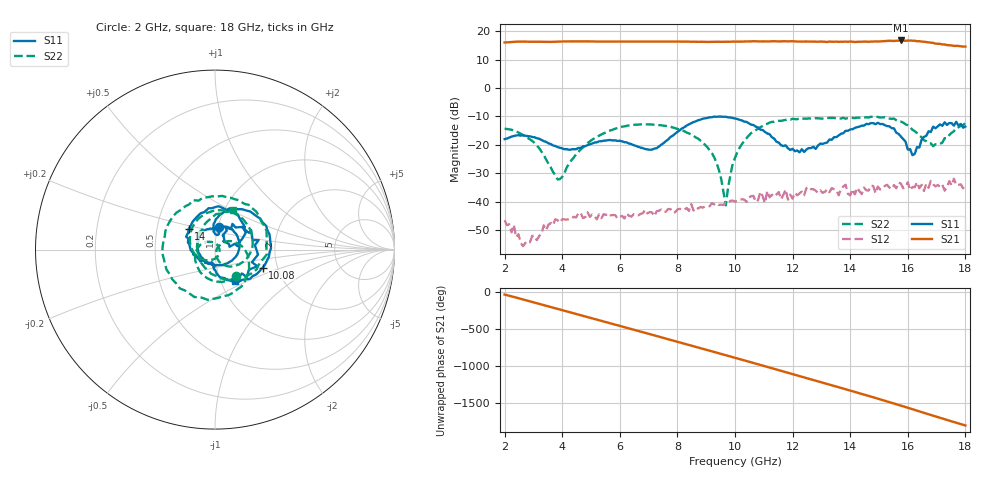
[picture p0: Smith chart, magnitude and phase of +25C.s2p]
!Agilent Technologies,N5230A,MY45001466,A.07.50.67
!Agilent N5230A: A.07.50.67
!Date: Monday, February 09, 2026 16:21:58
!Correction: S11(Full 2 Port(1,2))
!S21(Full 2 Port(1,2))
!S12(Full 2 Port(1,2))
!S22(Full 2 Port(1,2))
!S2P File: Measurements: S11, S21, S12, S22:
# Hz S  dB  R 50
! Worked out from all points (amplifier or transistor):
!   201 points, 2 GHz to 18 GHz, reference 50 ohm
!   highest |S21| = 16.7 dB at 15.76 GHz (marker M1)
!   |S21| within 3 dB of that: start of sweep to end of sweep
!   unconditionally stable (mu >= 1): start of sweep to end of sweep
!   at 4.64 GHz: K = 11.69, MAG = 16.5 dB, |S12| = -43.9 dB
!   at 10 GHz: K = 6.99, MAG = 16.7 dB, |S12| = -40.0 dB
!   at 18 GHz: K = 4.16, MAG = 15.1 dB, |S12| = -33.9 dB
!   S11 on the Smith chart (normalised r, x): 2 GHz: 1.01, +0.26; 10.08 GHz: 1.67, -0.37; 14 GHz: 0.73, +0.17; 18 GHz: 1.17, -0.43
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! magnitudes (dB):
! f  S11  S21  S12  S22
! 2 GHz  -18.0  16.0  -46.5  -14.4
! 2.64 GHz  -16.7  16.3  -55.6  -16.5
! 3.84 GHz  -20.8  16.3  -46.5  -32.2
! 4.72 GHz  -20.6  16.4  -45.7  -20.9
! 7.36 GHz  -20.6  16.3  -43.2  -13.0
! 9.04 GHz  -10.5  16.2  -41.6  -20.8
! 9.44 GHz  -10.0  16.2  -41.2  -28.8
! 9.68 GHz  -10.1  16.3  -40.4  -41.3
! 10 GHz  -10.7  16.3  -40.0  -24.6
! 10.08 GHz  -10.9  16.3  -39.7  -22.6
! 10.88 GHz  -14.6  16.4  -36.5  -13.8
! 11.04 GHz  -15.5  16.4  -40.5  -12.8
! 11.12 GHz  -16.0  16.4  -36.2  -12.6
! 11.92 GHz  -21.8  16.4  -37.5  -11.1
! 12.72 GHz  -20.7  16.3  -35.6  -10.8
! 13.84 GHz  -15.1  16.3  -34.0  -10.8
! 14 GHz  -14.6  16.4  -37.8  -10.6
! 15.36 GHz  -13.5  16.6  -35.0  -10.7
! 15.76 GHz  -17.1  16.7  -33.7  -11.8
! 16.16 GHz  -23.6  16.6  -34.8  -14.7
! 16.88 GHz  -13.6  15.8  -33.9  -20.5
! 18 GHz  -13.6  14.6  -33.9  -12.3
